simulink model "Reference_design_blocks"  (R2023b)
settings: Solver=VariableStepAuto  StartTime=0.0  StopTime=100.0  RelTol=1e-3
InitFcn:
  | PreprocIn0data  = dataPreProc('data/input_sig_i0.txt');
  | PreprocIn1data  = dataPreProc('data/input_sig_i1.txt');
  | PreprocOutdata  = dataPreProc('data/output_adder.txt');
undefined symbols (not defined in the file or in its folder): KernelClass, namespace, None
libraries: matrix_library x6, aieDSP x5, aieBasic x4, dspsrcs4 x3, aieUtilities x1

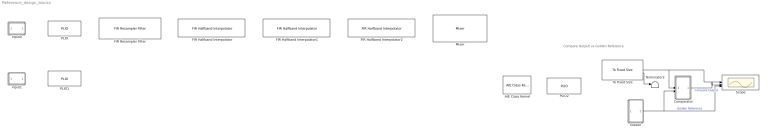
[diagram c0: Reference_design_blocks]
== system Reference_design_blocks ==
  note: Compare Output vs Golden Reference
  AIE Class Kernel : aieBasic/AIE Class Kernel  PortNames={}  PortSerializedTypes={}  PortWindowSizes={}  PortWindowMargins={}  PortSynchronicities={}  PortSignalSizes={}  ClassTemplateParamNames={}  ClassTemplateParamKinds={}  ClassTemplateParamTypes={}  ClassTemplateParamValues={}  ClassCtorParamNames={}  ClassCtorParamSerializedTypes={}  ClassCtorParamValues={}  ClassIndex=0  ClassCtorIndex=0  ClassTabVisible=off  ClassTemplateParamsVisible=off  ClassCtorDeclVisible=off  ClassCtorParamsVisible=off  FunctionTabVisible=off  PortAttrs={}  PortAttrsEnables=0  SampleTime=-1  ClassDeclTypeOptions=C[1 1]@t7@<empty>  ClassDecl=<empty>  ClassTemplateParams={}  ClassTemplateParamsEnables={}  ClassCtorDeclTypeOptions=C[1 1]@t7@<empty>  ClassCtorDecl=<empty>  ClassCtorParams={}  KernelClassName=namespace::KernelClass  KernelFunction=KernelFunction  KernelSearchPaths={}  PreProcOptions={}  blockJsonConstraints=[]
  Comparator : Subsystem
  FIR Halfband Interpolator : aieDSP/FIR Halfband Interpolator  data_type=cint16  coef_type=int16  use_coeff_reload=off  dual_ip=off  num_outputs=off  coeff=[-2,5,-9,17,-30,52,-98,316,500]  fir_length=31  input_window_size=256  shift_val=0  rnd_mode=Floor  sat_mode=0-None  interp_poly=1  upshift_ct=0  casc_length=1  AIE_VARIANT=1  blockJsonConstraints=[]  blockJsonConstraintsInternal=[]  spec=vmc_fir_interpolate_hb.json  SerializedMaskParamNames=[]  SerializedMaskParamValues=[]  SerializedMaskParamVisibilities=[]  block_type=FIR Halfband Interpolator  SerializedMaskParamDataypes=typename|typename|bool|bool|bool|coef_type|uint|uint|uint|uint|uint|uint|uint|uint|uint  SerializedMaskParamEnumStrArr=0|0|0|0|0|0|0|0|0|Floor,Ceiling,Round to positive infinity,Round to negative infinity,Round symmetrical to infinity,Round symmetrical to zero,Round convergent to even,Round convergent to odd|0-None,1-Asymmetric,3-Symmetric|0|0|0|0  SerializedMaskParamEnumValArr=0|0|0|0|0|0|0|0|0|0,1,2,3,4,5,6,7|0,1,3|0|0|0|0  SerializedMaskParamVectorArr=0|0|0|0|0|1|0|0|0|0|0|0|0|0|0
  FIR Halfband Interpolator1 : aieDSP/FIR Halfband Interpolator  data_type=cint16  coef_type=int16  use_coeff_reload=off  dual_ip=off  num_outputs=off  coeff=[-2,5,-9,17,-30,52,-98,316,500]  fir_length=31  input_window_size=256  shift_val=0  rnd_mode=Floor  sat_mode=0-None  interp_poly=1  upshift_ct=0  casc_length=1  AIE_VARIANT=1  blockJsonConstraints=[]  blockJsonConstraintsInternal=[]  spec=vmc_fir_interpolate_hb.json  SerializedMaskParamNames=[]  SerializedMaskParamValues=[]  SerializedMaskParamVisibilities=[]  block_type=FIR Halfband Interpolator  SerializedMaskParamDataypes=typename|typename|bool|bool|bool|coef_type|uint|uint|uint|uint|uint|uint|uint|uint|uint  SerializedMaskParamEnumStrArr=0|0|0|0|0|0|0|0|0|Floor,Ceiling,Round to positive infinity,Round to negative infinity,Round symmetrical to infinity,Round symmetrical to zero,Round convergent to even,Round convergent to odd|0-None,1-Asymmetric,3-Symmetric|0|0|0|0  SerializedMaskParamEnumValArr=0|0|0|0|0|0|0|0|0|0,1,2,3,4,5,6,7|0,1,3|0|0|0|0  SerializedMaskParamVectorArr=0|0|0|0|0|1|0|0|0|0|0|0|0|0|0
  FIR Halfband Interpolator2 : aieDSP/FIR Halfband Interpolator  data_type=cint16  coef_type=int16  use_coeff_reload=off  dual_ip=off  num_outputs=off  coeff=[-2,5,-9,17,-30,52,-98,316,500]  fir_length=31  input_window_size=256  shift_val=0  rnd_mode=Floor  sat_mode=0-None  interp_poly=1  upshift_ct=0  casc_length=1  AIE_VARIANT=1  blockJsonConstraints=[]  blockJsonConstraintsInternal=[]  spec=vmc_fir_interpolate_hb.json  SerializedMaskParamNames=[]  SerializedMaskParamValues=[]  SerializedMaskParamVisibilities=[]  block_type=FIR Halfband Interpolator  SerializedMaskParamDataypes=typename|typename|bool|bool|bool|coef_type|uint|uint|uint|uint|uint|uint|uint|uint|uint  SerializedMaskParamEnumStrArr=0|0|0|0|0|0|0|0|0|Floor,Ceiling,Round to positive infinity,Round to negative infinity,Round symmetrical to infinity,Round symmetrical to zero,Round convergent to even,Round convergent to odd|0-None,1-Asymmetric,3-Symmetric|0|0|0|0  SerializedMaskParamEnumValArr=0|0|0|0|0|0|0|0|0|0,1,2,3,4,5,6,7|0,1,3|0|0|0|0  SerializedMaskParamVectorArr=0|0|0|0|0|1|0|0|0|0|0|0|0|0|0
  FIR Resampler Filter : aieDSP/FIR Resampler Filter  data_type=cint16  coef_type=int16  use_coeff_reload=off  num_outputs=off  coeff=[1, zeros(1,29)]  fir_length=30  interpolate_factor=3  decimate_factor=2  input_window_size=256  shift_val=0  rnd_mode=Floor  sat_mode=0-None  interp_poly=1  deci_poly=1  casc_length=1  AIE_VARIANT=1  blockJsonConstraints=[]  blockJsonConstraintsInternal=[]  spec=vmc_fir_resampler.json  SerializedMaskParamNames=[]  SerializedMaskParamValues=[]  SerializedMaskParamVisibilities=[]  block_type=FIR Resampler Filter  SerializedMaskParamDataypes=typename|typename|bool|bool|coef_type|uint|uint|uint|uint|uint|uint|uint|uint|uint|uint|uint  SerializedMaskParamEnumStrArr=0|0|0|0|0|0|0|0|0|0|Floor,Ceiling,Round to positive infinity,Round to negative infinity,Round symmetrical to infinity,Round symmetrical to zero,Round convergent to even,Round convergent to odd|0-None,1-Asymmetric,3-Symmetric|0|0|0|0  SerializedMaskParamEnumValArr=0|0|0|0|0|0|0|0|0|0|0,1,2,3,4,5,6,7|0,1,3|0|0|0|0  SerializedMaskParamVectorArr=0|0|0|0|1|0|0|0|0|0|0|0|0|0|0|0
  Golden : Subsystem
  Mixer : aieDSP/Mixer  data_type=cint16  input_window_size=32  rnd_mode=Floor  sat_mode=0-None  mixer_mode=Single Input Mode  USE_PHASE_RELOAD=off  phase_increment=0  AIE_VARIANT=1  blockJsonConstraints=[]  blockJsonConstraintsInternal=[]  spec=vmc_mixer.json  SerializedMaskParamNames=[]  SerializedMaskParamValues=[]  SerializedMaskParamVisibilities=[]  block_type=Mixer  SerializedMaskParamDataypes=typename|uint|uint|uint|uint|bool|uint|uint  SerializedMaskParamEnumStrArr=0|0|Floor,Ceiling,Round to positive infinity,Round to negative infinity,Round symmetrical to infinity,Round symmetrical to zero,Round convergent to even,Round convergent to odd|0-None,1-Asymmetric,3-Symmetric|Single Input Mode,Dual Input Mode|0|0|0  SerializedMaskParamEnumValArr=0|0|0,1,2,3,4,5,6,7|0,1,3|1,2|0|0|0  SerializedMaskParamVectorArr=0|0|0|0|0|0|0|0
  PLIO : aieBasic/PLIO  PlioWidth=auto  PlioFreqSpec=off  PlioFreq=250  ColLocation=0  channel=0  blockJsonConstraints=[]  deprecateConstraints=0
  PLIO1 : aieBasic/PLIO  PlioWidth=auto  PlioFreqSpec=off  PlioFreq=250  ColLocation=0  channel=0  blockJsonConstraints=[]  deprecateConstraints=0
  PLIO2 : aieBasic/PLIO  PlioWidth=auto  PlioFreqSpec=off  PlioFreq=250  ColLocation=0  channel=0  blockJsonConstraints=[]  deprecateConstraints=0
  Scope : Scope  NumInputPorts=3
  Terminator2 : Terminator
  To Fixed Size : aieUtilities/To Fixed Size  Mode=Produce a valid output signal  OutputSize=3072  CopyMethod=Buffer samples to form output  HasStatusOutput=on
  input0 : Subsystem
  input1 : Subsystem
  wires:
  Golden/1(Out1) -> Comparator/2(In2), Scope/3  "Golden Reference"
  Comparator/1(Out1) -> Scope/2  "Compare Output"
  To Fixed Size/1 -> Scope/1, Comparator/1(In1)
  To Fixed Size/2 -> Terminator2/1

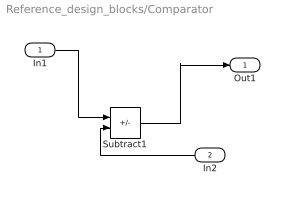
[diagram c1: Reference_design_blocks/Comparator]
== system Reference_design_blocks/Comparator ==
  In1 : Inport
  In2 : Inport  Port=2
  Subtract1 : Sum  Inputs=+-  OutDataTypeStr=double
  Out1 : Outport
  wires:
  In1/1 -> Subtract1/1
  In2/1 -> Subtract1/2
  Subtract1/1 -> Out1/1

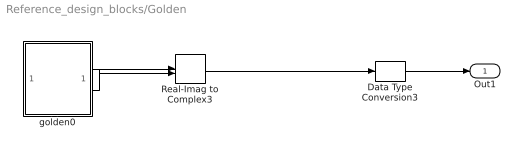
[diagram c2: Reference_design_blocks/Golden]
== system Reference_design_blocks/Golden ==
  Data Type Conversion3 : DataTypeConversion  OutDataTypeStr=int16
  Real-Imag to Complex3 : RealImagToComplex
  golden0 : Subsystem
  Out1 : Outport
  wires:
  Real-Imag to Complex3/1 -> Data Type Conversion3/1
  golden0/2(Out2) -> Real-Imag to Complex3/2
  golden0/1(Out1) -> Real-Imag to Complex3/1
  Data Type Conversion3/1 -> Out1/1

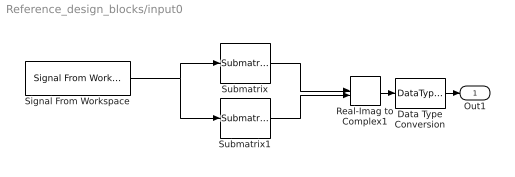
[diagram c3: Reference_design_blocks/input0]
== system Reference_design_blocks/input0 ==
  Data Type Conversion : DataTypeConversion  OutDataTypeStr=int16
  Real-Imag to Complex1 : RealImagToComplex
  Signal From Workspace : dspsrcs4/Signal From Workspace  X=PreprocIn0data  Ts=1  nsamps=256  OutputAfterFinalValue=Setting to zero  ignoreOrWarnInputAndFrameLengths=off  OutputFrames=off
  Submatrix : matrix_library/Submatrix  RowSpan=All rows  RowStartMode=First  RowStartIndex=1  RowEndMode=Last  RowEndIndex=1  ColSpan=One column  ColStartMode=First  ColStartIndex=1  ColEndMode=Last  ColEndIndex=1
  Submatrix1 : matrix_library/Submatrix  RowSpan=All rows  RowStartMode=First  RowStartIndex=1  RowEndMode=Last  RowEndIndex=1  ColSpan=One column  ColStartMode=Last  ColStartIndex=1  ColEndMode=Last  ColEndIndex=1
  Out1 : Outport
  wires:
  Signal From Workspace/1 -> Submatrix1/1, Submatrix/1
  Submatrix/1 -> Real-Imag to Complex1/1
  Submatrix1/1 -> Real-Imag to Complex1/2
  Real-Imag to Complex1/1 -> Data Type Conversion/1
  Data Type Conversion/1 -> Out1/1

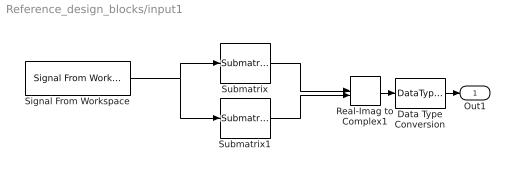
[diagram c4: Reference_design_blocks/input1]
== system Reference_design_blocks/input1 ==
  Data Type Conversion : DataTypeConversion  OutDataTypeStr=int16
  Real-Imag to Complex1 : RealImagToComplex
  Signal From Workspace : dspsrcs4/Signal From Workspace  X=PreprocIn1data  Ts=1  nsamps=256  OutputAfterFinalValue=Setting to zero  ignoreOrWarnInputAndFrameLengths=off  OutputFrames=off
  Submatrix : matrix_library/Submatrix  RowSpan=All rows  RowStartMode=First  RowStartIndex=1  RowEndMode=Last  RowEndIndex=1  ColSpan=One column  ColStartMode=First  ColStartIndex=1  ColEndMode=Last  ColEndIndex=1
  Submatrix1 : matrix_library/Submatrix  RowSpan=All rows  RowStartMode=First  RowStartIndex=1  RowEndMode=Last  RowEndIndex=1  ColSpan=One column  ColStartMode=Last  ColStartIndex=1  ColEndMode=Last  ColEndIndex=1
  Out1 : Outport
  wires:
  Signal From Workspace/1 -> Submatrix1/1, Submatrix/1
  Submatrix/1 -> Real-Imag to Complex1/1
  Submatrix1/1 -> Real-Imag to Complex1/2
  Real-Imag to Complex1/1 -> Data Type Conversion/1
  Data Type Conversion/1 -> Out1/1

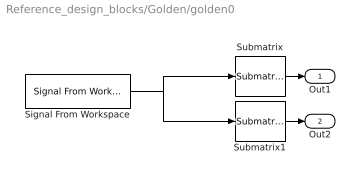
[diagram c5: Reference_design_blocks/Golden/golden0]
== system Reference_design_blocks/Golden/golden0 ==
  Signal From Workspace : dspsrcs4/Signal From Workspace  X=PreprocOutdata  Ts=1  nsamps=3072  OutputAfterFinalValue=Setting to zero  ignoreOrWarnInputAndFrameLengths=on  OutputFrames=off
  Submatrix : matrix_library/Submatrix  RowSpan=All rows  RowStartMode=First  RowStartIndex=1  RowEndMode=Last  RowEndIndex=1  ColSpan=One column  ColStartMode=First  ColStartIndex=1  ColEndMode=Last  ColEndIndex=1
  Submatrix1 : matrix_library/Submatrix  RowSpan=All rows  RowStartMode=First  RowStartIndex=1  RowEndMode=Last  RowEndIndex=1  ColSpan=One column  ColStartMode=Last  ColStartIndex=1  ColEndMode=Last  ColEndIndex=1
  Out1 : Outport  VectorParamsAs1DForOutWhenUnconnected=off
  Out2 : Outport  Port=2  VectorParamsAs1DForOutWhenUnconnected=off
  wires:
  Submatrix/1 -> Out1/1
  Signal From Workspace/1 -> Submatrix/1, Submatrix1/1
  Submatrix1/1 -> Out2/1
